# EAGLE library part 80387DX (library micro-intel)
MICROCOMPUTER/PERIPHERAL DEVICE
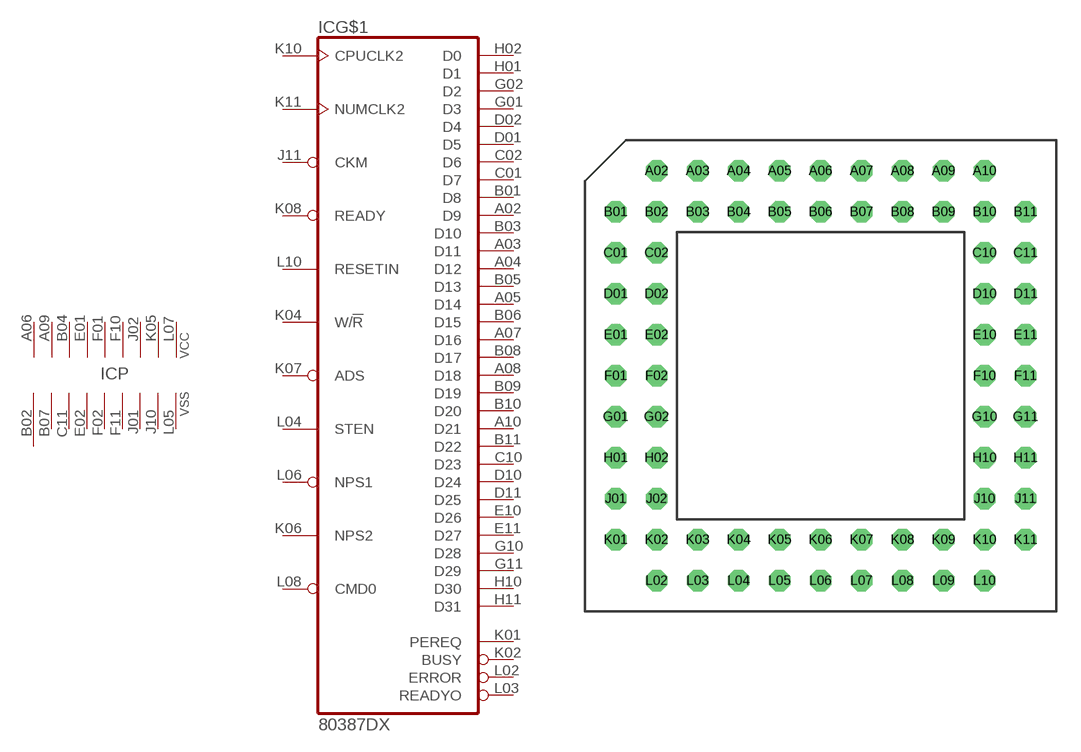
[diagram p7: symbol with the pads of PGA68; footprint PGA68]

Designator prefix IC; gates G$1=80387DX P=9VCC9VSS

## 80387DX (OC_FARNELL: unknown; OC_NEWARK: unknown)  [PGA68]
A02  G$1:D9
A03  G$1:D11
A04  G$1:D12
A05  G$1:D14
A06  P:VCC  pwr
A07  G$1:D16
A08  G$1:D18
A09  P:VCC  pwr
A10  G$1:D21
B01  G$1:D8
B02  P:VSS  pwr
B03  G$1:D10
B04  P:VCC  pwr
B05  G$1:D13
B06  G$1:D15
B07  P:VSS  pwr
B08  G$1:D17
B09  G$1:D19
B10  G$1:D20
B11  G$1:D22
C01  G$1:D7
C02  G$1:D6
C10  G$1:D23
C11  P:VSS  pwr
D01  G$1:D5
D02  G$1:D4
D10  G$1:D24
D11  G$1:D25
E01  P:VCC  pwr
E02  P:VSS  pwr
E10  G$1:D26
E11  G$1:D27
F01  P:VCC  pwr
F02  P:VSS  pwr
F10  P:VCC  pwr
F11  P:VSS  pwr
G01  G$1:D3
G02  G$1:D2
G10  G$1:D28
G11  G$1:D29
H01  G$1:D1
H02  G$1:D0
H10  G$1:D30
H11  G$1:D31
J01  P:VSS  pwr
J02  P:VCC  pwr
J10  P:VSS  pwr
J11  G$1:CKM  in
K01  G$1:PEREQ  out
K02  G$1:BUSY  out
K04  G$1:W/!R  in
K05  P:VCC  pwr
K06  G$1:NPS2  in
K07  G$1:ADS  in
K08  G$1:READY  in
K10  G$1:CPUCLK2  in
K11  G$1:NUMCLK2  in
L02  G$1:ERROR  out
L03  G$1:READYO  out
L04  G$1:STEN  in
L05  P:VSS  pwr
L06  G$1:NPS1  in
L07  P:VCC  pwr
L08  G$1:CMD0  in
L10  G$1:RESETIN  in

## Footprint PGA68 (pad centres in mm)
Pin Grid Array
drill 0.813 octagon: A02 -10.16,12.7; A03 -7.62,12.7; A04 -5.08,12.7; A05 -2.54,12.7; A06 0,12.7; A07 2.54,12.7; A08 5.08,12.7; A09 7.62,12.7; A10 10.16,12.7; B01 -12.7,10.16; B02 -10.16,10.16; B03 -7.62,10.16; B04 -5.08,10.16; B05 -2.54,10.16; B06 0,10.16; B07 2.54,10.16; B08 5.08,10.16; B09 7.62,10.16; B10 10.16,10.16; B11 12.7,10.16; C01 -12.7,7.62; C02 -10.16,7.62; C10 10.16,7.62; C11 12.7,7.62; D01 -12.7,5.08; D02 -10.16,5.08; D10 10.16,5.08; D11 12.7,5.08; E01 -12.7,2.54; E02 -10.16,2.54; E10 10.16,2.54; E11 12.7,2.54; F01 -12.7,0; F02 -10.16,0; F10 10.16,0; F11 12.7,0; G01 -12.7,-2.54; G02 -10.16,-2.54; G10 10.16,-2.54; G11 12.7,-2.54; H01 -12.7,-5.08; H02 -10.16,-5.08; H10 10.16,-5.08; H11 12.7,-5.08; J01 -12.7,-7.62; J02 -10.16,-7.62; J10 10.16,-7.62; J11 12.7,-7.62; K01 -12.7,-10.16; K02 -10.16,-10.16; K03 -7.62,-10.16; K04 -5.08,-10.16; K05 -2.54,-10.16; K06 0,-10.16; K07 2.54,-10.16; K08 5.08,-10.16; K09 7.62,-10.16; K10 10.16,-10.16; K11 12.7,-10.16; L02 -10.16,-12.7; L03 -7.62,-12.7; L04 -5.08,-12.7; L05 -2.54,-12.7; L06 0,-12.7; L07 2.54,-12.7; L08 5.08,-12.7; L09 7.62,-12.7; L10 10.16,-12.7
